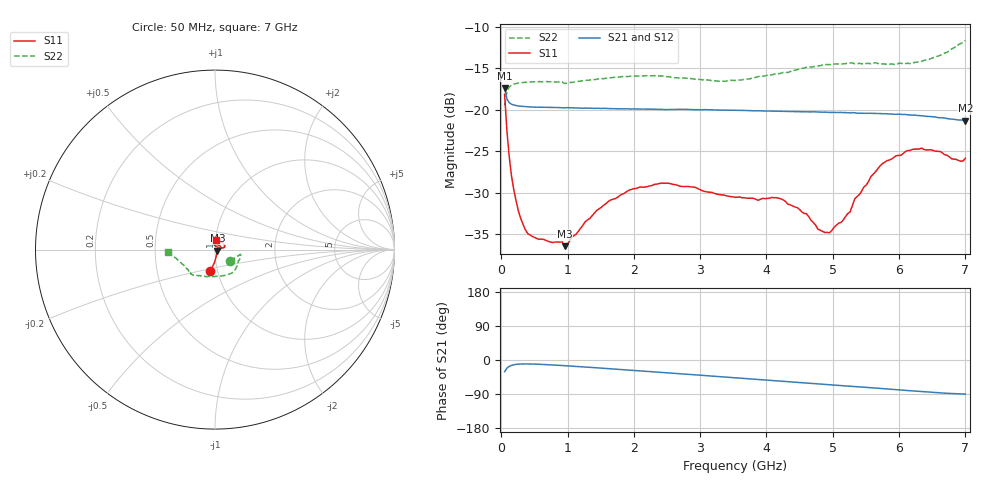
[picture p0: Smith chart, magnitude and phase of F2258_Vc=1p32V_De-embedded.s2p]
! Integrated Device Technology
! Corporate Headquarters
! 6024 Silver Creek Valley Road
! San Jose, CA 95138  USA
! Phone:  1-408-284-8200
! Toll Free:  1-800-223-1366
! Webpage:  http://www.idt.com/
! Timing and RF Division
! 515 Groton Road, Suite 102
! Westford, MA 01886-6024
! Device:  F2258
! Description: Voltage Variable RF Attenuator
! Frequency:  50.0 -  6000.00 MHz
! Package:  3x3 mm Thin QFN Plastic Package: 16 pin
! Ports:  2 RF, 2 DC
!  Pin  1  = NC
!  Pin  2  = NC
!  Pin  3  = RF2  = Port 2
!  Pin  4  = GND
!  Pin  5  = Vdd
!  Pin  6  = NC
!  Pin  7  = VCTRL
!  Pin  8  = NC
!  Pin  9  = GND
!  Pin 10  = RF1  = Port 1
!  Pin 11  = NC
!  Pin 12  = NC
!  Pin 13  = NC
!  Pin 14  = NC
!  Pin 15  = NC
!  Pin 16  = NC
! Vcntrl:  1.320 Volts
! Vdd:  +3.300 Volts
! Current:  1.165 mA
! Data:  The device was measured on a the F2258 evaluation board which has
!  individual transmission lines to the RF pins.  Data was collected
!  using a calibrated network analyzer.  The evaluation board was
!  de-embedded using a TRL calibration technique.
!  The reference plane is the edge of the package pin.
! Misc:  SN 10
!  Action Tracker AT0285
! Date Measured:  2014-12-10
! Date:  2016-01-13  MJV
! Note:
!  Integrated Device Technology supplies this data as a sample of measured
!  data at the package pin for this product.  Your particular data for this
!  product may vary.
!  Data was taken at 25 degrees C.
!  Integrated Device Technology reserves the right to change this data at anytime.
!Freq_(GHz)  S11M_(dB)  S11P_(deg)  S21M_(dB)  S21P_(deg)  S12M_(dB)  S12P_(deg)  S22M_(dB)  S22P_(deg)
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# GHz S dB R 50
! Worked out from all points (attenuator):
!   201 points, 50 MHz to 7 GHz, reference 50 ohm
!   highest |S21| = -17.38 dB at 50 MHz (marker M1); lowest = -21.3 dB at 7 GHz (marker M2)
!   lowest |S11| = -36.4 dB at 953.5 MHz (marker M3), VSWR 1.03, Z = 51.4 - j0.641 ohm
!   |S11| at or under -10 dB: start of sweep to end of sweep
!   |S22| runs from -19.5 to -11.7 dB; largest |S21 - S12| = 0.00084
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0.05  -18.11 -102.2  -17.38 -30.7  -17.34 -30.6  -19.47 -36.3
0.08475  -22.54 -93.3  -18.69 -21.5  -18.64 -21.4  -17.82 -17.5
0.15425  -27.96 -81.4  -19.33 -14.1  -19.28 -14.1  -17.04 -11.6
0.22375  -31.00 -71.5  -19.49 -11.6  -19.45 -11.6  -16.84 -10.5
0.29325  -33.09 -60.6  -19.58 -10.6  -19.53 -10.6  -16.74 -11.3
0.43225  -35.06 -44.3  -19.66 -10.5  -19.61 -10.5  -16.65 -13.3
0.9535  -36.41 -24.3  -19.77 -14.9  -19.71 -14.9  -16.84 -25.5
1.2315  -33.88 -9.2  -19.81 -18.1  -19.76 -18.1  -16.49 -32.1
1.6485  -30.86 -0.0  -19.86 -23.2  -19.82 -23.2  -16.15 -41.1
2.37825  -28.88 18.5  -19.94 -32.2  -19.91 -32.2  -15.92 -56.8
3.525  -30.53 71.8  -20.07 -46.9  -20.05 -47.0  -16.47 -94.2
4.22  -30.72 98.9  -20.19 -55.9  -20.20 -55.9  -15.60 -118.0
4.60225  -32.49 94.1  -20.24 -60.7  -20.25 -60.7  -14.88 -126.3
4.7065  -33.56 85.1  -20.24 -62.2  -20.24 -62.2  -14.83 -127.8
4.94975  -34.79 57.4  -20.32 -65.2  -20.31 -65.2  -14.56 -130.8
5.2625  -32.27 24.2  -20.37 -69.2  -20.38 -69.2  -14.36 -134.2
5.332  -30.71 19.7  -20.36 -70.2  -20.38 -70.1  -14.46 -134.5
5.57525  -28.03 12.7  -20.42 -73.2  -20.43 -73.2  -14.46 -137.9
5.85325  -26.04 12.8  -20.50 -76.9  -20.52 -76.8  -14.51 -142.2
6.33975  -24.61 22.5  -20.73 -83.4  -20.78 -83.3  -14.17 -154.3
6.9305  -26.18 73.3  -21.23 -89.5  -21.25 -89.5  -12.03 -173.9
7  -25.83 84.0  -21.30 -89.8  -21.33 -89.8  -11.66 -176.5
